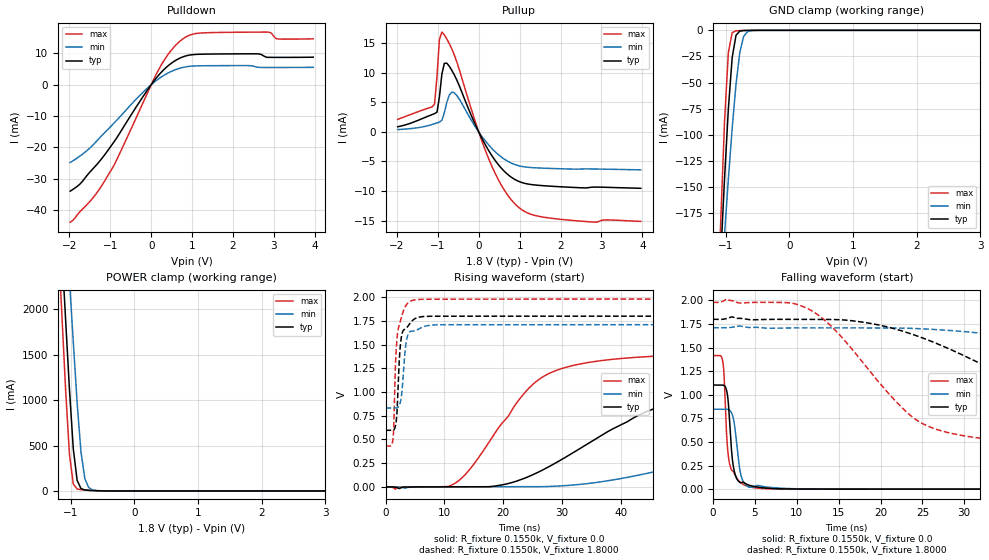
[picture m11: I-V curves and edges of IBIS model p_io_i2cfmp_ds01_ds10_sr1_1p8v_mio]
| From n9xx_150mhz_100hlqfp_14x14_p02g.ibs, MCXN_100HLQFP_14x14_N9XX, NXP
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[Model] p_io_i2cfmp_ds01_ds10_sr1_1p8v_mio
|   Model p_io_i2cfmp_ds01_ds10_sr1_1p8v_mio
| This model was characterised for following simulation conditions:
| External (pad) voltage:
|   - Typ: 1.8V,   - Min: 1.71V,   - Max: 1.98V
| Library cells for typ/min/max conditions are connected as defined below:
|  pad - External Pad
|  ipp_do_lv - Core Input
|  ipp_obe_lv - Output Buffer Enable
|  IOGC - NC
|  REFH3V3 - REFH3V3
|  REFL3V3 - REFL3V3
|  ZI - NC
|  abut_ncal_vddio[1] - vssio vddio vddio
|  abut_ncal_vddio[2] - vddio vddio vssio
|  abut_ncal_vddio[3] - vddio
|  abut_ncal_vddio[4] - vssio vddio vddio
|  abut_ncal_vddio[5] - vddio vddio vssio
|  abut_ncal_vddio[6] - vddio
|  abut_pcal_vddio[1] - vssio
|  abut_pcal_vddio[2] - vddio vssio vddio
|  abut_pcal_vddio[3] - vssio
|  abut_pcal_vddio[4] - vssio
|  abut_pcal_vddio[5] - vddio vssio vddio
|  abut_pcal_vddio[6] - vssio
|  ipp_do_1p8v - ipp_do_1p8v
|  ipp_dse_lv[0] - vdd_lv
|  ipp_dse_lv[1] - 0
|  ipp_eftd_lv - NC
|  ipp_ina_mux_vddio - NC
|  ipp_ina_mux_vddio[0] - NC
|  ipp_ina_mux_vddio[1] - NC
|  ipp_ina_r0_vddio - NC
|  ipp_ina_r0a_vddio - NC
|  ipp_ina_r0b_vddio - NC
|  ipp_ina_r0c_vddio - NC
|  ipp_ina_r0d_vddio - NC
|  ipp_ina_r0e_vddio - NC
|  ipp_ina_r0f_vddio - NC
|  ipp_ina_r300_vddio - NC
|  ipp_ina_r300a_vddio - NC
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Model_type I/O
Polarity   Non-Inverting
Enable   Active-High
Vinl =   0.5400V
Vinh =   1.2600V
Vmeas =  0.9000V
Cref =   30.0000pF
Rref =   1.0000M
Vref =   1.8000V
C_comp   1.7515pF   1.7218pF   1.7928pF
|C_comp_pullup   0.7571pF   0.8227pF   0.7008pF
|C_comp_pulldown   0.8805pF   0.8511pF   0.9098pF
[Model Spec]
| variable   typ   min   max
Vinh   1.2600V   1.1970V   1.3860V
Vinl   0.5400V   0.5130V   0.5940V
[Temperature Range]   25.0000   0.1250k   -40.0000
[Voltage Range]   1.8000V   1.7100V   1.9800V
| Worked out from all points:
|   slope of the pulldown table from 0 to 0.27 V, typ, clamps not added: 62.9 ohm
|   slope of the pullup table from 0 to 0.27 V, typ, clamps not added: 78.2 ohm
|   GND clamp passes 1 mA (typ) near -0.78 V on its own axis
|   POWER clamp passes 1 mA (typ) near -0.53 V on its own axis
|   rising waveform, R_fixture 0.1550k, V_fixture 0.0: 20-80 % time 20.7ns typ, 38.7ns min, 10.5ns max; typ from 0 V to 1.1 V
|   rising waveform, R_fixture 0.1550k, V_fixture 1.8000: 20-80 % time 652ps typ, 743ps min, 730ps max; typ from 0.596 V to 1.8 V
|   falling waveform, R_fixture 0.1550k, V_fixture 0.0: 20-80 % time 613ps typ, 708ps min, 585ps max; typ from 1.1 V to 0 V
|   falling waveform, R_fixture 0.1550k, V_fixture 1.8000: 20-80 % time 19.1ns typ, 37.2ns min, 9.44ns max; typ from 1.8 V to 0.596 V
[Pulldown]
|Voltage   I(typ)   I(min)   I(max)
-1.98V    -34.05mA   -24.87mA   -43.96mA
-1.74V    -31.75mA   -22.8mA    -40.58mA
-1.14V    -22.47mA   -15.36mA   -30.83mA
-900mV    -18.11mA   -12.15mA   -25.55mA
180mV     3.015mA    1.868mA    4.762mA
480mV     6.746mA    4.183mA    10.85mA
780mV     8.923mA    5.533mA    14.69mA
1.2V      9.737mA    6.042mA    16.51mA
2.58V     9.872mA    5.631mA    16.81mA
2.82V     8.763mA    5.507mA    16.82mA
3.06V     8.728mA    5.506mA    14.68mA
3.96V     8.792mA    5.545mA    14.66mA
[Pullup]
|Voltage   I(typ)   I(min)   I(max)
-1.98V    874.2uA    394.3uA    2.123mA
-1.08V    3.084mA    1.378mA    4.713mA
-1.02V    3.333mA    1.519mA    9.342mA
-960mV    5.93mA     1.665mA    15.68mA
-900mV    9.793mA    1.958mA    16.88mA
-840mV    11.6mA     3.244mA    16.41mA
-780mV    11.62mA    4.985mA    15.73mA
-600mV    9.684mA    6.632mA    13.07mA
240mV     -3.119mA   -2.177mA   -4.482mA
900mV     -8.107mA   -5.556mA   -12.28mA
1.74V     -9.17mA    -6.172mA   -14.57mA
3.96V     -9.537mA   -6.417mA   -15.13mA
[GND_clamp]
|Voltage   I(typ)   I(min)   I(max)
-1.98V    -1.571A    -1.243A    -2.046A
-1.14V    -296.8mA   -307.7mA   -291.9mA
-1.08V    -217.1mA   -250.6mA   -183.3mA
-1.02V    -142mA     -195.3mA   -87.29mA
-960mV    -75.42mA   -142.6mA   -21.4mA
-900mV    -26.21mA   -93.87mA   -2.23mA
-840mV    -4.776mA   -51.84mA   -446.5uA
-780mV    -725.4uA   -21.22mA   -243.9uA
-720mV    -200uA     -5.88mA    -159.3uA
-660mV    -98.47uA   -1.291mA   -98.82uA
-420mV    -3.926uA   -10.95uA   -2.45uA
3.96V     0A         0A         0A
[POWER_clamp]
|Voltage   I(typ)   I(min)   I(max)
-1.98V    13.51A     13.25A     14.01A
-1.2V     3.414A     4.356A     2.802A
-1.14V    2.644A     3.675A     1.949A
-1.08V    1.876A     2.995A     1.103A
-1.02V    1.113A     2.317A     397.9mA
-960mV    462.1mA    1.641A     75.38mA
-900mV    117mA      972.3mA    21.31mA
-840mV    26.38mA    432.6mA    13.76mA
-780mV    10.65mA    139.4mA    9.996mA
-720mV    6.506mA    38.48mA    6.892mA
-660mV    4.142mA    12.01mA    4.303mA
3.96V     0A         0A         0A
[Ramp]
| variable   typ   min   max
dV/dt_r  0.6621/20.6703n   0.5060/38.6842n   0.8497/10.5408n
dV/dt_f  0.7223/19.0955n   0.5248/37.1702n   0.9298/9.4384n
R_load = 0.1550k
[Rising Waveform]
R_fixture= 0.1550k
V_fixture= 0.0
V_fixture_min= 0.0
V_fixture_max= 0.0
|time   V(typ)   V(min)   V(max)
0s        874.6pV    404.1nV    21.73pV
11.55ns   -66.99uV   -36.23uV   29.6mV
19.24ns   14.72mV    1.592uV    627.5mV
25.46ns   140.7mV    503.2uV    1.105V
38.2ns    598.5mV    68.24mV    1.343V
46.43ns   842mV      170.2mV    1.38V
55.97ns   968.8mV    316.6mV    1.399V
73.09ns   1.051V     566.2mV    1.412V
93.16ns   1.084V     719.3mV    1.415V
212.3ns   1.103V     843.4mV    1.416V
[Rising Waveform]
R_fixture= 0.1550k
V_fixture= 1.8000
V_fixture_min= 1.7100
V_fixture_max= 1.9800
|time   V(typ)   V(min)   V(max)
0s        596mV      831.1mV    430.4mV
1.263ns   596.3mV    831.1mV    506.2mV
1.395ns   600.3mV    831.1mV    638.7mV
1.696ns   647.5mV    830.8mV    1.32V
2.179ns   1.13V      842.5mV    1.673V
2.459ns   1.452V     881.2mV    1.735V
2.826ns   1.621V     1.033V     1.814V
3.647ns   1.681V     1.57V      1.929V
5.205ns   1.78V      1.651V     1.974V
212.3ns   1.8V       1.71V      1.98V
[Falling Waveform]
R_fixture= 0.1550k
V_fixture= 0.0
V_fixture_min= 0.0
V_fixture_max= 0.0
|time   V(typ)   V(min)   V(max)
0s        1.103V     846.9mV    1.416V
1.177ns   1.104V     846.6mV    1.344V
1.317ns   1.099V     847mV      1.201V
1.694ns   1.012V     847.5mV    472.8mV
2.12ns    512.3mV    822.1mV    219.4mV
2.6ns     167.9mV    655.6mV    153.2mV
3.11ns    78.16mV    252.9mV    84.03mV
3.481ns   72.9mV     105.8mV    56.33mV
5.582ns   18.56mV    35.89mV    8.813mV
212.3ns   229.3nV    3.234uV    46.01nV
[Falling Waveform]
R_fixture= 0.1550k
V_fixture= 1.8000
V_fixture_min= 1.7100
V_fixture_max= 1.9800
|time   V(typ)   V(min)   V(max)
0s        1.8V       1.71V      1.98V
11.08ns   1.8V       1.709V     1.923V
14.38ns   1.798V     1.71V      1.704V
24.16ns   1.63V      1.702V     741.3mV
35.28ns   1.183V     1.621V     510.3mV
42.46ns   905.2mV    1.529V     474.8mV
50.64ns   760.9mV    1.399V     454.8mV
70.36ns   653.5mV    1.087V     437mV
89.36ns   620.7mV    956.1mV    432.4mV
212.3ns   596.2mV    835.4mV    430.4mV
